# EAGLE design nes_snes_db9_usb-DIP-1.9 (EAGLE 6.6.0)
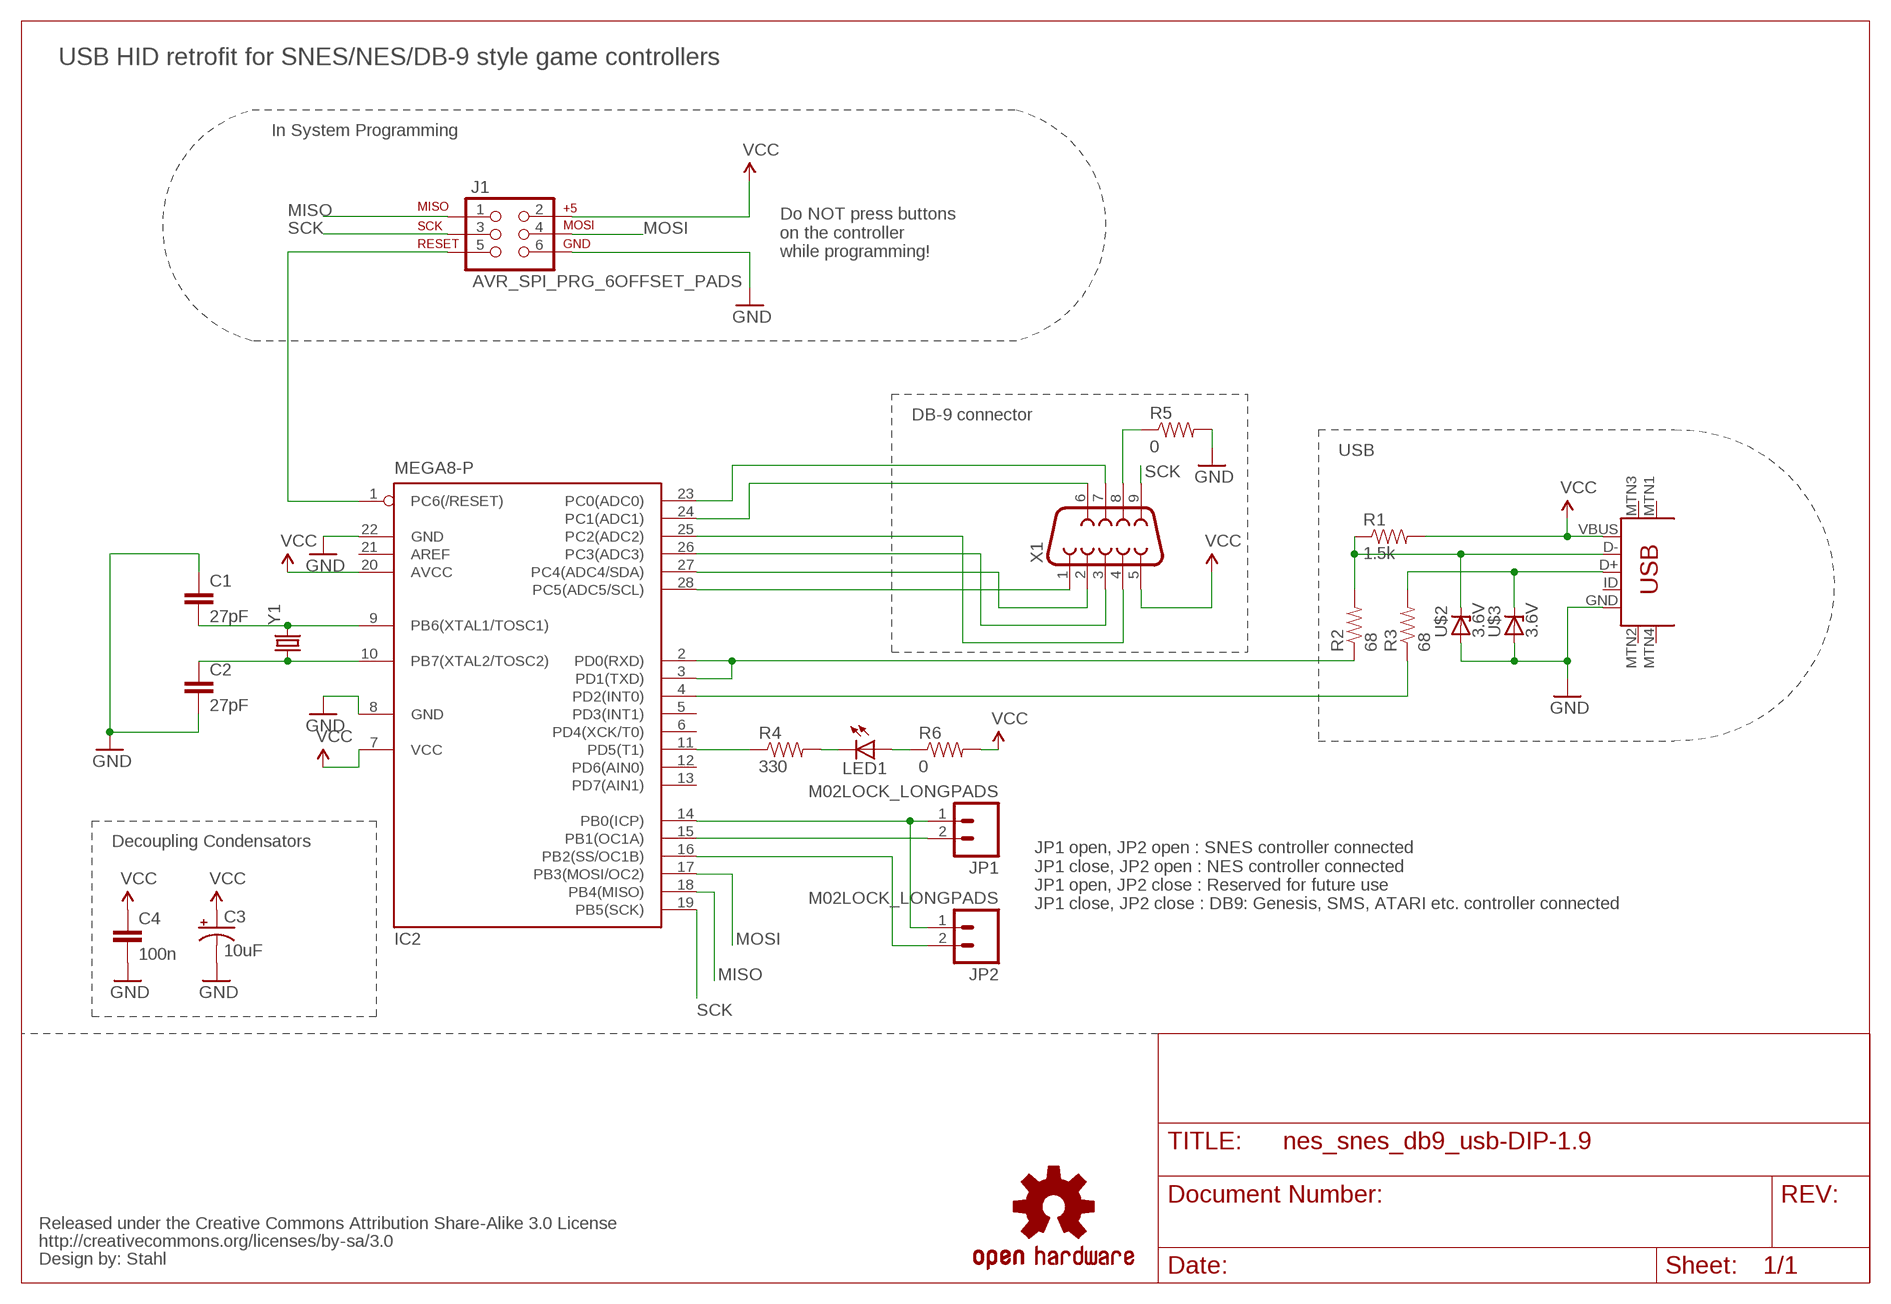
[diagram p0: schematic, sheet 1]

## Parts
C1  27pF  CAP1206  [1206]
C2  27pF  CAP1206  [1206]
C3  10uF  CPOL-USB  [PANASONIC_B]
C4  100n  CAP1206  [1206]
CC_TEXT1  CREATIVE_COMMONS  [CREATIVE_COMMONS]
IC2  MEGA8-P  [DIL28-3]
J1  AVR_SPI_PRG_6OFFSET_PADS  [2X3_OFFSET]
JP1  M02LOCK_LONGPADS  [1X02_LOCK_LONGPADS]
JP2  M02LOCK_LONGPADS  [1X02_LOCK_LONGPADS]
LED1  LED1206  [LED-1206]
LOGO1  OSHW-LOGOL  [OSHW-LOGO-L]
R1  1.5k  RESISTOR1206  [1206]
R2  68  RESISTOR1206  [1206]
R3  68  RESISTOR1206  [1206]
R4  330  RESISTOR1206  [1206]
R5  0  RESISTOR1206  [1206]
R6  0  RESISTOR1206  [1206]
U$1  USB-MINIB-5PIN  [USB-MINIB]
U$2  3.6V  ZENER-DIODESOD80C  [SOD80C]
U$3  3.6V  ZENER-DIODESOD80C  [SOD80C]
X1  DB9MALE  [DB9_MALE]
Y1  CRYSTALSMD  [HC49UP]

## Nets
D+: R3.2 U$1.D+ U$3.C
D-: R1.1 R2.2 U$1.D- U$2.C
GND: C1.1 C2.2 C3.- C4.2 IC2.8(GND) IC2.22(GND) J1.6 R5.2 U$1.GND U$2.A U$3.A
MISO: IC2.18(PB4(MISO)) J1.1
MOSI: IC2.17(PB3(MOSI/OC2)) J1.4
N$1: R5.1 X1.8
N$2: C1.2 IC2.9(PB6(XTAL1/TOSC1)) Y1.2
N$3: C2.1 IC2.10(PB7(XTAL2/TOSC2)) Y1.1
N$4: IC2.11(PD5(T1)) R4.1
N$5: LED1.C R4.2
N$6: IC2.14(PB0(ICP)) JP1.1 JP2.1
N$7: IC2.15(PB1(OC1A)) JP1.2
N$8: IC2.16(PB2(SS/OC1B)) JP2.2
N$9: LED1.A R6.1
N$10: IC2.2(PD0(RXD)) IC2.3(PD1(TXD)) R2.1
N$12: IC2.4(PD2(INT0)) R3.1
N$13: IC2.28(PC5(ADC5/SCL)) X1.1
N$14: IC2.27(PC4(ADC4/SDA)) X1.2
N$15: IC2.26(PC3(ADC3)) X1.3
N$16: IC2.25(PC2(ADC2)) X1.4
N$18: IC2.24(PC1(ADC1)) X1.6
N$19: IC2.23(PC0(ADC0)) X1.7
RESET: IC2.1(PC6(/RESET)) J1.5
SCK: IC2.19(PB5(SCK)) J1.3 X1.9
VCC: C3.+ C4.1 IC2.7(VCC) IC2.20(AVCC) J1.2 R1.2 R6.2 U$1.VBUS X1.5
Unconnected: IC2.5(PD3(INT1)) IC2.6(PD4(XCK/T0)) IC2.12(PD6(AIN0)) IC2.13(PD7(AIN1)) IC2.21(AREF) U$1.ID U$1.MTN1(MTN2) U$1.MTN2(MTN3) U$1.MTN3(MTN1) U$1.MTN4

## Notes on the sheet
- USB HID retrofit for SNES/NES/DB-9 style game controllers
- In System Programming
- Do NOT press buttons
  on the controller
  while programming!
- DB-9 connector
- USB
- Decoupling Condensators
- JP1 open, JP2 open : SNES controller connected
  JP1 close, JP2 open : NES controller connected
  JP1 open, JP2 close : Reserved for future use
  JP1 close, JP2 close : DB9: Genesis, SMS, ATARI etc. controller connected

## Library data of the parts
C1 C2 C4 = SparkFun-Capacitors:CAP: Capacitor
C3 = adafruit:CPOL-US: POLARIZED CAPACITOR, American symbol
CC_TEXT1 = SparkFun-Aesthetics:CREATIVE_COMMONS: Creative Commons License summary
IC2 = atmel:MEGA8-P: MICROCONTROLLER 8 Kbytes FLASH, 1 kbytes SRAM, 512 bytes EEPROM, USART, 4-channel 10 bit ADC, 2-channel 8 bit ADC Pin compatible with Atmega48, ATMega88, ATMega168 Source: avr.lbr; OC_FARNELL: unknown; OC_NEWARK: unknown
J1 = SparkFun-Connectors:AVR_SPI_PRG_6: AVR ISP 6 Pin This is the reduced ISP connector for AVR programming. Common on Arduino. This footprint will take up less PCB space and can be used with a 10-pin to 6-pin adapter such as SKU: BOB-08508
JP1 JP2 = SparkFun-Connectors:M02: Standard 2-pin 0.1" header. Use with
LED1 = SparkFun-LED:LED: LEDs
LOGO1 = SparkFun-Aesthetics:OSHW-LOGO: Open Source Hardware Logo This logo indicates the piece of hardware it is found on incorporates a OSHW license and/or adheres to the definition of open source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
R1-R6 = SparkFun-Resistors:RESISTOR: Resistor
U$1 = SparkFun-Connectors:USB-MINIB: Mini-USB "B" connector with 5th pin broken out. Created new symbol breaking out 5th "ID" pin in mini/micro USB connector spec. See: http://en.wikipedia.org/wiki/Mini_usb#Cables. Uses same footprint as 4-pin symbol. Also added pins to connect to mounting / shield pads if required (probably not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
U$2 U$3 = diode:ZENER-DIODE: Z-Diode
X1 = SparkFun-Connectors:DB9: DB9 Connector Standard DB9 (D-Sub 9) serial connector. Can be used for CAN bus as well as RS485 and RS232. Footprint production proven. Spark Fun Electronics SKU : PRT-00429
Y1 = SparkFun-FreqCtrl:CRYSTAL: Various standard crystals. Proven footprints. Spark Fun Electronics SKU : COM-00534

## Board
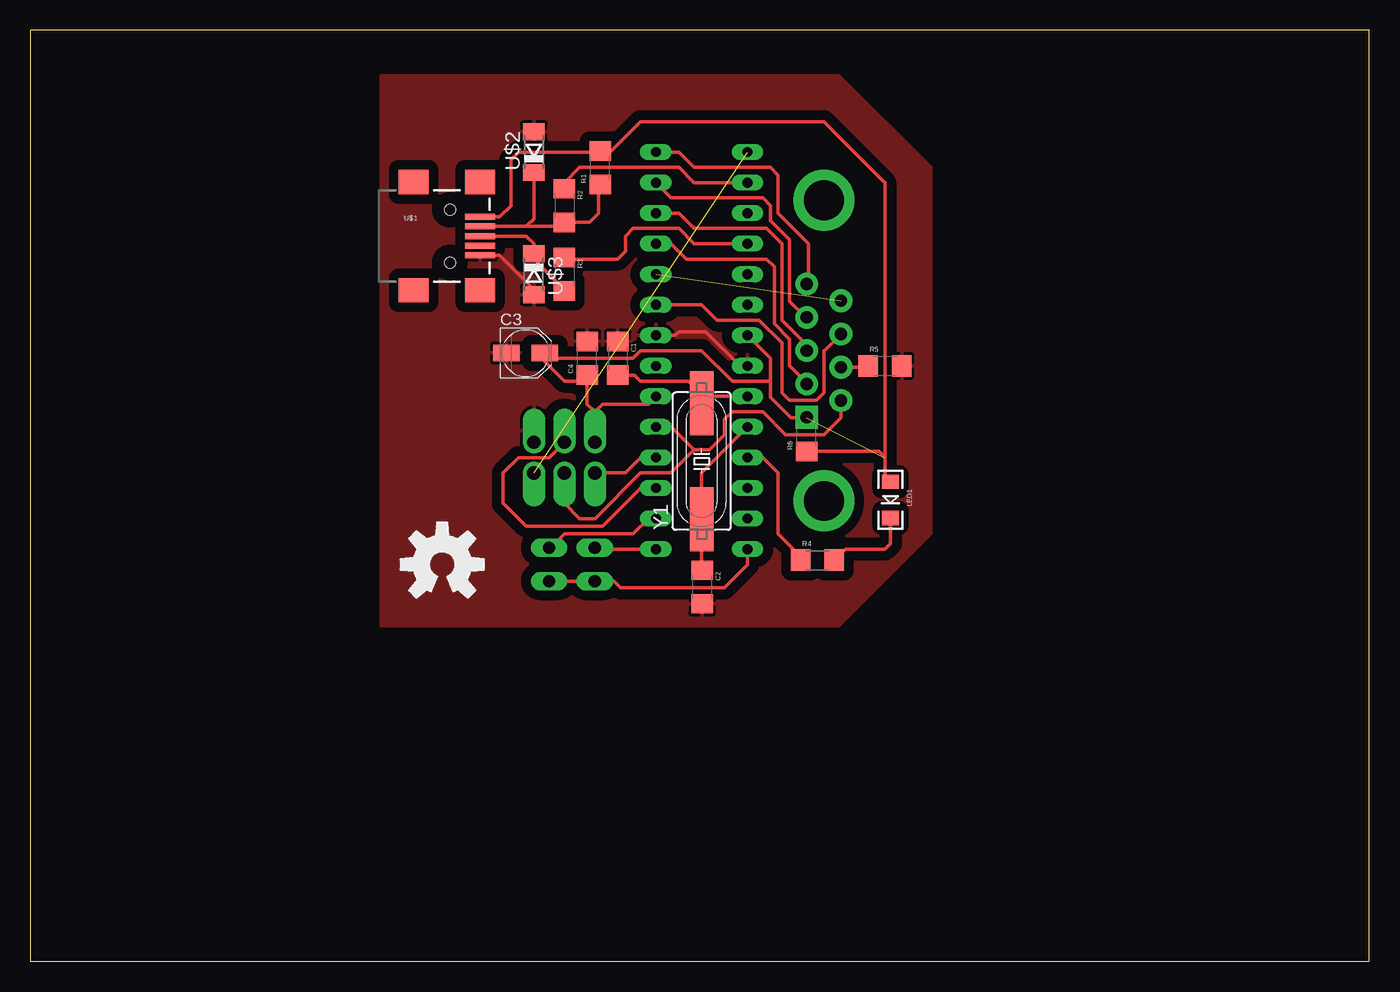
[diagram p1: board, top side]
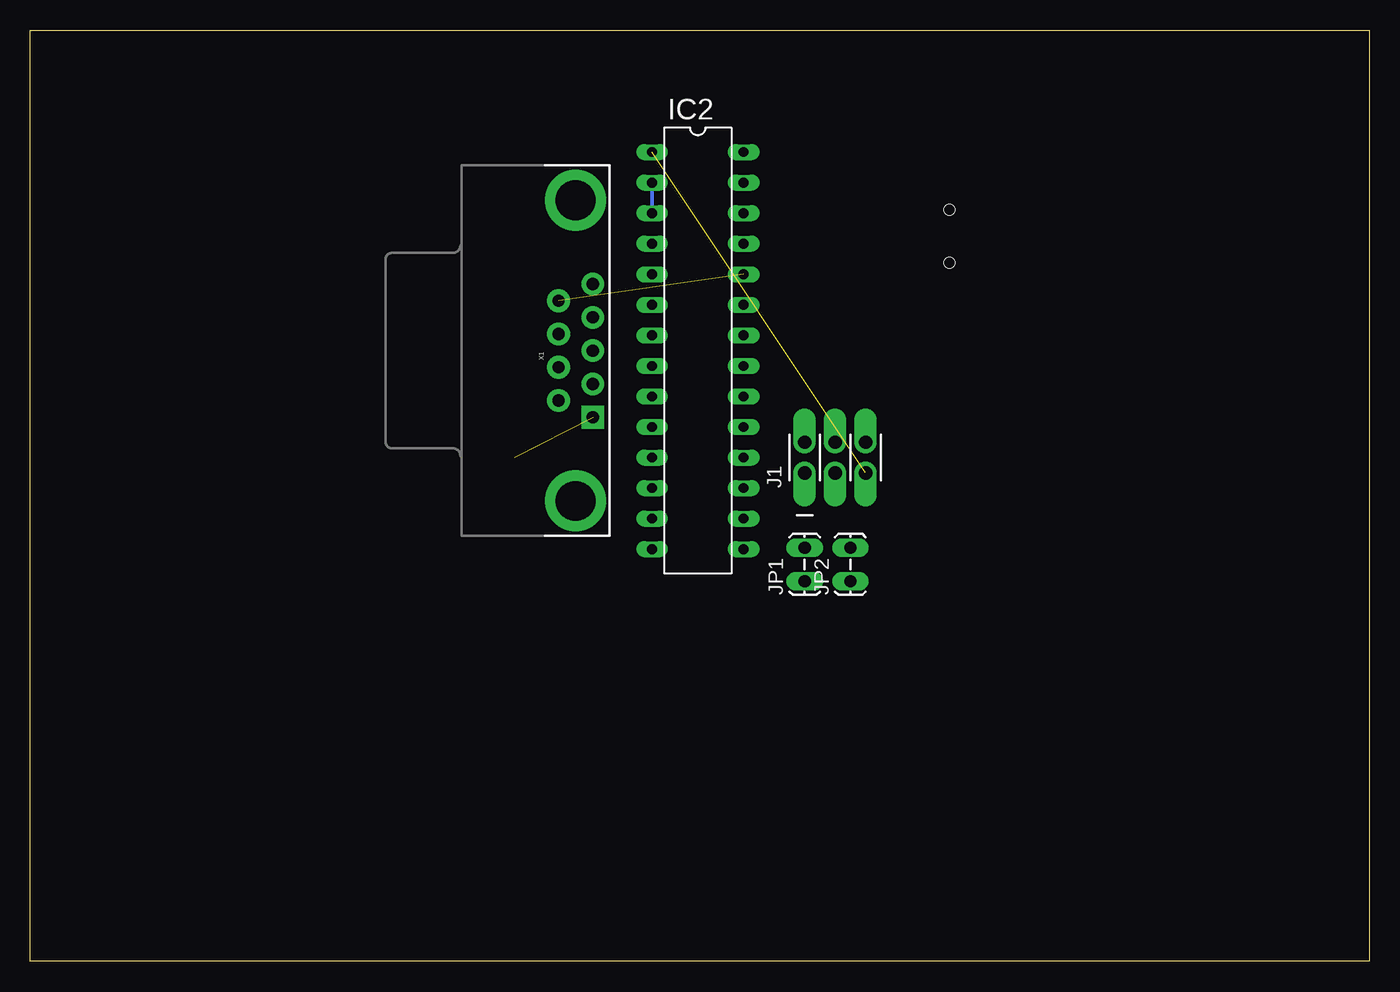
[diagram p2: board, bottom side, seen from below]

Size 111.43 x 77.46 mm. Coordinates in mm from the lower left corner, seen from the top.
Outline: 0,0 111.43,0 111.43,77.46 0,77.46 0,0
Copper layers (1*16): Top 0.035mm / dielectric 1.5mm / Bottom 0.035mm
Design rules "default": minimum track width 10mil, minimum drill 24mil, track to track 8mil, track to pad 8mil, pad to pad 8mil, via to via 8mil, smd to smd 8mil, copper to edge 40mil, drill to drill 8mil, minimum pad ring 10mil, minimum via ring 8mil, stop-mask expansion 4mil, vias tented up to drill 0mil, thermal gap 10mil

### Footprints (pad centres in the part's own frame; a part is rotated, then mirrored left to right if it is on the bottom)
1206 = smd 1.6 x 1.8: 1 -1.4,0; 2 1.4,0
PANASONIC_B = smd 2.2 x 1.4: + 1.6,0; - -1.6,0
DIL28-3 = drill 0.813 long: 1 -16.51,-3.81; 2 -13.97,-3.81; 3 -11.43,-3.81; 4 -8.89,-3.81; 5 -6.35,-3.81; 6 -3.81,-3.81; 7 -1.27,-3.81; 8 1.27,-3.81; 9 3.81,-3.81; 10 6.35,-3.81; 11 8.89,-3.81; 12 11.43,-3.81; 13 13.97,-3.81; 14 16.51,-3.81; 15 16.51,3.81; 16 13.97,3.81; 17 11.43,3.81; 18 8.89,3.81; 19 6.35,3.81; 20 3.81,3.81; 21 1.27,3.81; 22 -1.27,3.81; 23 -3.81,3.81; 24 -6.35,3.81; 25 -8.89,3.81; 26 -11.43,3.81; 27 -13.97,3.81; 28 -16.51,3.81
2X3_OFFSET = drill 1.118 pad 1.88 offset: 1 -2.54,-1.27; 2 -2.54,1.27; 3 0,-1.27; 4 0,1.27; 5 2.54,-1.27; 6 2.54,1.27
1X02_LOCK_LONGPADS = drill 1.016 long: 1 -0.127,0; 2 2.667,0
LED-1206 = smd 1.2 x 1.4: A -1.5,0; C 1.5,0
USB-MINIB = smd 2.5 x 0.5: D+ 2.5,0; D- 2.5,0.8; GND 2.5,-1.6; ID 2.5,-0.8; VBUS 2.5,1.6 | smd 2.5 x 2: MTN1 -3,4.5; MTN2 2.5,4.5; MTN3 -3,-4.5; MTN4 2.5,-4.5 | hole 0.9: 0,2.2; 0,-2.2
SOD80C = smd 1.4 x 1.8: A 1.7,0; C -1.7,0
DB9_MALE = drill 1.016 pad 1.88: 1 5.54,-1.42; 2 2.77,-1.42; 3 0,-1.42; 4 -2.77,-1.42; 6 4.15,1.42; 7 1.38,1.42; 8 -1.38,1.42; 9 -4.15,1.42 | drill 1.016 pad 1.88 square: 5 -5.54,-1.42 | drill 3.302 pad 5.08: G1 -12.5,0; G2 12.5,0
HC49UP = smd 5.334 x 1.93: 1 -4.826,0; 2 4.826,0

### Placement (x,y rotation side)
C1  48.9,50.16 270 top
C2  55.91,31.14 270 top
C3  41.23,50.6 0 top
C4  46.35,50.16 90 top
CC_TEXT1  22.86,2.54 0 top
IC2  55.88,50.8 270 bottom
J1  44.45,41.91 0 bottom
JP1  46.99,31.75 90 bottom
JP2  43.18,31.75 90 bottom
LED1  71.59,38.4 270 top
LOGO1  34.29,33.02 0 top
R1  47.43,66.01 90 top
R2  44.45,62.87 270 top
R3  44.45,57.15 270 top
R4  65.51,33.38 0 top
R5  71.12,49.53 0 top
R6  64.6,43.82 90 top
U$1  34.92,60.32 0 top
U$2  41.91,67.31 90 top
U$3  41.91,57.15 270 top
X1  66.04,50.8 90 bottom
Y1  55.88,41.6 90 top

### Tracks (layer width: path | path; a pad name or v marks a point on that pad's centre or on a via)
D+
  Top 0.305: R3.2 44.45,55.88 41.91,58.42 U$3.C 41.91,59.69 41.27,60.32 U$1.D+
D-
  Top 0.305: U$1.D- 41.27,61.12 | 41.27,61.12 44.11,61.12 R2.2 46.54,61.46 47.31,62.23 47.31,64.49 R1.1 | U$2.C 41.91,61.76 41.27,61.12
GND
  Top 0.305: U$1.GND 39.06,58.73 41.91,55.88 42.34,55.88 U$3.A | IC2.8 59.05,49.53 56.2,52.39 53.98,52.39 53.66,52.07 IC2.22
  pour Top (isolate 0.813): 29.21,73.66 67.31,73.66 74.93,66.04 74.93,35.56 67.31,27.94 29.21,27.94
MISO
  Top 0.305: J1.1 49.53,40.64 50.8,41.91 IC2.18
MOSI
  Top 0.305: J1.4 43.18,41.91 40.64,41.91 39.37,40.64 39.37,38.1 41.27,36.2 47.62,36.2 50.8,39.37 IC2.17
N$1
  Top 0.305: X1.8 69.61,49.42 R5.1
N$2
  Top 0.305: Y1.2 56.1,46.95 | 56.1,46.95 56.12,47.07 56.2,46.99 IC2.9 | C1.2 50.3,48.77 50.8,48.26 54.79,48.26 56.1,46.95
N$3
  Top 0.305: C2.1 55.88,33.21 Y1.1 55.88,40.64 IC2.10
N$4
  Top 0.305: R4.1 64.11,33.68 62.23,35.56 62.23,40.64 60.96,41.91 IC2.11
N$5
  Top 0.305: LED1.C 71.59,34.76 71.12,34.29 67.83,34.29 R4.2
N$6
  Top 0.305: JP2.1 JP1.1 48.57,31.62 49.12,31.06 57.77,31.06 59.7,33 IC2.14
N$7
  Top 0.305: JP1.2 46.86,34.42 46.99,34.29 IC2.15
N$8
  Top 0.305: JP2.2 43.31,34.42 44.45,35.56 50.16,35.56 51.44,36.83 IC2.16
N$9
  Top 0.305: R6.1 70.61,42.42 71.12,41.91 71.12,40.36 LED1.A
N$10
  Top 0.305: IC2.2 55.24,64.77 53.98,66.04 45.72,66.04 44.45,64.77 R2.1
  Bottom 0.305: IC2.2 IC2.3
N$12
  Top 0.305: R3.1 44.45,58.42 48.9,58.42 49.53,59.05 49.53,60.32 50.16,60.96 53.98,60.96 55.24,59.69 IC2.4
N$13
  Top 0.305: X1.1 64.94,56.34 64.77,56.52 64.77,59.69 62.23,62.23 62.23,65.41 61.59,66.04 55.24,66.04 53.98,67.31 IC2.28
N$14
  Top 0.305: X1.2 64.54,53.57 63.18,54.93 63.18,60.01 61.59,61.59 61.59,62.87 60.96,63.5 53.34,63.5 IC2.27
N$15
  Top 0.305: X1.3 64.67,51.22 62.55,53.34 62.55,59.69 61.28,60.96 55.24,60.96 53.98,62.23 IC2.26
N$16
  Top 0.305: X1.4 64.36,48.35 63.18,49.53 63.18,51.75 61.91,53.02 61.91,57.78 61.28,58.42 54.61,58.42 53.34,59.69 IC2.25
N$18  (1 unrouted)
N$19
  Top 0.305: IC2.23 55.88,54.61 57.15,53.34 60.64,53.34 62.55,51.44 62.55,47.31 63.18,46.67 65.41,46.67 66.04,47.31 66.04,50.8 66.08,50.8 X1.7
RESET  (1 unrouted)
SCK
  Top 0.305: X1.9 67.46,45.23 66.04,43.81 62.87,43.81 60.96,45.72 58.42,45.72 57.78,45.08 57.78,43.81 56.52,42.55 55.24,42.55 | J1.3 44.45,38.1 45.72,36.83 46.99,36.83 50.8,40.64 53.34,40.64 55.24,42.55 | IC2.19 53.34,44.45 55.24,42.55
VCC  (1 unrouted)
  Top 0.305: 61.59,48.26 61.59,50.16 IC2.7 | U$1.VBUS 39.06,61.92 40.01,62.87 40.01,66.67 40.64,67.31 47.33,67.31 R1.2 48.36,67.41 50.8,69.85 66.04,69.85 71.12,64.77 71.12,41.91 | C4.1 46.35,48.26 | 46.35,48.26 46.35,46.35 46.99,45.72 | 46.99,45.72 J1.2 | 46.99,45.72 47.62,46.35 51.44,46.35 IC2.20 | 46.35,48.26 44.45,48.26 42.84,49.88 C3.+ 43.27,50.16 50.16,50.16 50.8,50.8 55.88,50.8 58.42,48.26 61.59,48.26 | 61.59,48.26 61.59,46.91 63.3,45.2 64.56,45.2 X1.5 64.56,45.26 R6.2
